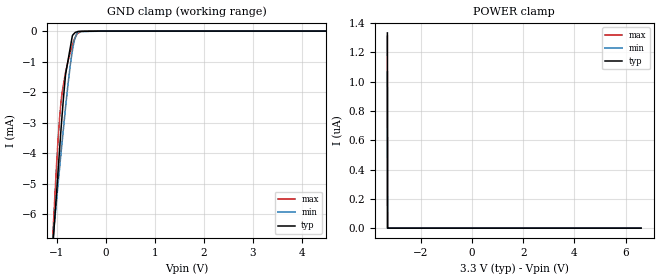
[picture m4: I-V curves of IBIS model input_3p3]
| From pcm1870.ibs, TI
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|   input_3p3 Model
[Model]   input_3p3
Model_type   Input
Vinl = 0.99
Vinh = 2.31
|   typ   min   max
C_comp   5.013e-13   4.599e-13   5.301e-13
[Model spec]
Vinl   0.99   0.9   1.08
Vinh   2.31   2.1   2.52
[Voltage Range]   3.3   3   3.6
|Ambient Temperature   25   85   -40
|Junction Temperature
[Temperature Range]   26   86   -40
[Power Clamp Reference]   3.3   3   3.6
[GND Clamp Reference]   0   0   0
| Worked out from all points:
|   GND clamp passes 1 mA (typ) near -0.78 V on its own axis
[GND Clamp]
|   Voltage   I(typ)   I(min)   I(max)
-3.3V     -60.52mA   -45.86mA   -82.36mA
-1.089V   -7.173mA   -6.948mA   -6.84mA
-1.056V   -6.377mA   -6.374mA   -5.794mA
-978mV    -4.592mA   -5.015mA   -3.561mA
-942mV    -3.769mA   -4.402mA   -2.752mA
-895.2mV  -2.752mA   -3.637mA   -2.012mA
-825mV    -1.424mA   -2.496mA   -1.357mA
-686.4mV  -156.2uA   -652.2uA   -454uA
-627mV    -44.46uA   -210.4uA   -209.9uA
-537mV    -9.471uA   -16.27uA   -37.49uA
-391.2mV  -6.342uA   -10.74uA   -26.9nA
6.6V      0A         0A         0A
[POWER Clamp]
|   Voltage   I(typ)   I(min)   I(max)
-3.3V     1.334uA    1.063uA    1.312uA
-3.294V   121.2nA    0A         218.6nA
-3.293V   0A         0A         109.3nA
-3.293V   0A         0A         0A
6.6V      0A         0A         0A
